| TEXAS INSTRUMENTS INCORPORATED
| Standard Linear and Logic Group
| IBIS Model of SN74LVC823A
| 9-Bit Bus-Interface Flip-Flop with 3-State Outputs
| This file contains package information for the following:
|  TSSOP 24-pin (PW) package as [Component] LVC823A_PW
|  SSOP 24-pin (DB) package as [Component] LVC823A_DB
|  TVSOP 24-pin (DGV) package as [Component] LVC823A_DGV
|  SOIC 24-pin (DW) package as [Component] LVC823A_DW
|  SOP 24-pin (NS) package as [Component] LVC823A_NS
| This device can be powered at the following Vccs:
|  1.8 volt Vcc
|  2.5 volt Vcc
|  3.3 volt Vcc
| This file provides unique models under the [Model Selector] for each Vcc.
| For operation at a specific Vcc, select the appropriate model after each
| [Model Selector] keyword.
[IBIS Ver]   3.2
[Comment char]  |_char
[File Name]   sn74lvc823a.ibs
[File Rev]   1.1 | a
[Date]   May 6, 2005
[Source]   Data created from TI-SPICE simulations at TI-SLL.
[Notes]   The following is an IBIS list for the LVC823A.
   Please contact sllibis@ti.com with questions and
   comments concerning SLL IBIS models.
   This IBIS model is created from a BA (back annotated netlist)
   - FILE REV HISTORY
   - 1.1 Release IBIS file on 05/06/05
   - Power-clamp data has been deleted since there is no
   power-clamp diode in the device.
   - Due to the fact that the device is 5-V input/output
   tolerant, the pullup data has some non-monotonic warnings.
   - End point warning due to AC and DC mismatch.
[Disclaimer] Property of Texas Instruments Incorporated.  Unauthorized
   reproduction and/or distribution is strictly prohibited.
   This product is protected under copyright law.
   Created  2005, (C) Copyright  2005, Texas Instruments
   Incorporated, All Rights Reserved
   UNLESS THERE IS A SIGNED, WRITTEN AGREEMENT TO THE
   CONTRARY, TEXAS INSTRUMENTS (TI) IS PROVIDING THE IBIS
   MODELS  AND WITHOUT ANY WARRANTY, EXPRESSED OR
   IMPLIED.  TI assumes no liability for:
   1) the accuracy of the IBIS models provided to your
   company;
   2) the proper functioning of these IBIS Models in your
   design or for any resulting applications; or
   3) infringement of patents, copyrights or intellectual
   property rights resulting from your use of these IBIS
   models.
   TI provides IBIS Models as a service to our customers.
   You and your company shall not distribute, sell or give
   these models to anyone else without prior written
   permission from TI.
   TI reserves the right to make changes to our products or
   to discontinue any semiconductor product or service
   without notice, and advises our customers to obtain the
   latest version of relevant information to verify, before
   placing orders, that the information being relied on is
   current.
   Please be aware that your receipt and use of the IBIS
   information provided shall serve as acceptance of these
   terms and conditions.  If you do not accept these terms,
   you should return or destroy the IBIS models and any
   other accompanying information immediately.
| Component LVC823A_PW 24-pin TSSOP
[Component]   LVC823A_PW
[Manufacturer]   Texas Instruments, Inc.
[Package]
|   typ   min   max
R_pkg   3.900e-02   3.000e-02   4.600e-02
L_pkg   2.685e-09   2.367e-09   3.177e-09
C_pkg   3.200e-13   2.520e-13   4.340e-13
[Pin]   signal_name   model_name   R_pin   L_pin   C_pin
1   NOE   LVC823A_NOE   3.700e-02   3.153e-09   4.340e-13
2   1D   LVC823A_IN   3.400e-02   2.629e-09   3.410e-13
3   2D   LVC823A_IN   3.200e-02   2.860e-09   3.470e-13
4   3D   LVC823A_IN   4.200e-02   2.741e-09   2.900e-13
5   4D   LVC823A_IN   4.600e-02   2.600e-09   2.620e-13
6   5D   LVC823A_IN   4.300e-02   2.414e-09   2.660e-13
7   6D   LVC823A_IN   4.200e-02   2.367e-09   2.620e-13
8   7D   LVC823A_IN   4.400e-02   2.461e-09   2.520e-13
9   8D   LVC823A_IN   4.200e-02   2.543e-09   2.740e-13
10   9D   LVC823A_IN   3.000e-02   2.616e-09   3.320e-13
11   NCLR   LVC823A_NCLR   3.700e-02   2.670e-09   3.460e-13
12   GND   GND   3.900e-02   3.177e-09   4.330e-13
13   CLK   LVC823A_CLK   3.700e-02   3.111e-09   4.310e-13
14   NCLKEN   LVC823A_NCLKEN   3.700e-02   2.656e-09   3.450e-13
15   9Q   LVC823A_OUT   3.100e-02   2.739e-09   3.400e-13
16   8Q   LVC823A_OUT   4.200e-02   2.649e-09   2.820e-13
17   7Q   LVC823A_OUT   4.600e-02   2.532e-09   2.570e-13
18   6Q   LVC823A_OUT   4.400e-02   2.425e-09   2.660e-13
19   5Q   LVC823A_OUT   4.400e-02   2.425e-09   2.660e-13
20   4Q   LVC823A_OUT   4.600e-02   2.532e-09   2.570e-13
21   3Q   LVC823A_OUT   4.200e-02   2.648e-09   2.820e-13
22   2Q   LVC823A_OUT   3.100e-02   2.738e-09   3.390e-13
23   1Q   LVC823A_OUT   3.600e-02   2.653e-09   3.440e-13
24   VCC   POWER   3.700e-02   3.110e-09   4.310e-13
| Component LVC823A_DB 24-pin SSOP
[Component]   LVC823A_DB
[Manufacturer]   Texas Instruments, Inc.
[Package]
|   typ   min   max
R_pkg   4.500e-02   4.000e-02   4.900e-02
L_pkg   3.668e-09   3.226e-09   4.415e-09
C_pkg   4.160e-13   3.490e-13   5.070e-13
[Pin]   signal_name   model_name   R_pin   L_pin   C_pin
1   NOE   LVC823A_NOE   4.200e-02   4.299e-09   5.030e-13
2   1D   LVC823A_IN   4.000e-02   3.960e-09   4.990e-13
3   2D   LVC823A_IN   4.200e-02   3.775e-09   4.170e-13
4   3D   LVC823A_IN   4.700e-02   3.487e-09   3.690e-13
5   4D   LVC823A_IN   4.600e-02   3.347e-09   3.520e-13
6   5D   LVC823A_IN   4.900e-02   3.352e-09   3.710e-13
7   6D   LVC823A_IN   4.600e-02   3.226e-09   3.630e-13
8   7D   LVC823A_IN   4.700e-02   3.289e-09   3.490e-13
9   8D   LVC823A_IN   4.700e-02   3.347e-09   3.610e-13
10   9D   LVC823A_IN   4.100e-02   3.576e-09   4.090e-13
11   NCLR   LVC823A_NCLR   4.100e-02   3.995e-09   5.030e-13
12   GND   GND   4.500e-02   4.415e-09   5.070e-13
13   CLK   LVC823A_CLK   4.300e-02   4.337e-09   5.060e-13
14   NCLKEN   LVC823A_NCLKEN   4.200e-02   4.003e-09   5.040e-13
15   9Q   LVC823A_OUT   4.100e-02   3.686e-09   4.100e-13
16   8Q   LVC823A_OUT   4.800e-02   3.355e-09   3.490e-13
17   7Q   LVC823A_OUT   4.700e-02   3.301e-09   3.530e-13
18   6Q   LVC823A_OUT   4.800e-02   3.268e-09   3.660e-13
19   5Q   LVC823A_OUT   4.800e-02   3.269e-09   3.660e-13
20   4Q   LVC823A_OUT   4.700e-02   3.314e-09   3.490e-13
21   3Q   LVC823A_OUT   4.800e-02   3.399e-09   3.550e-13
22   2Q   LVC823A_OUT   4.100e-02   3.688e-09   4.120e-13
23   1Q   LVC823A_OUT   4.200e-02   4.003e-09   5.040e-13
24   VCC   POWER   4.300e-02   4.347e-09   5.050e-13
| Component LVC823A_DGV 24-pin TVSOP
[Component]   LVC823A_DGV
[Manufacturer]   Texas Instruments, Inc.
[Package]
|   typ   min   max
R_pkg   4.300e-02   3.900e-02   4.700e-02
L_pkg   2.601e-09   2.312e-09   3.626e-09
C_pkg   3.580e-13   2.770e-13   5.950e-13
[Pin]   signal_name   model_name   R_pin   L_pin   C_pin
1   NOE   LVC823A_NOE   4.300e-02   3.625e-09   5.950e-13
2   1D   LVC823A_IN   4.000e-02   2.656e-09   4.020e-13
3   2D   LVC823A_IN   3.900e-02   2.338e-09   3.080e-13
4   3D   LVC823A_IN   4.600e-02   2.354e-09   2.770e-13
5   4D   LVC823A_IN   4.500e-02   2.312e-09   2.850e-13
6   5D   LVC823A_IN   4.700e-02   2.318e-09   2.820e-13
7   6D   LVC823A_IN   4.700e-02   2.318e-09   2.820e-13
8   7D   LVC823A_IN   4.500e-02   2.312e-09   2.850e-13
9   8D   LVC823A_IN   4.600e-02   2.353e-09   2.780e-13
10   9D   LVC823A_IN   3.900e-02   2.338e-09   3.080e-13
11   NCLR   LVC823A_NCLR   4.100e-02   2.660e-09   4.020e-13
12   GND   GND   4.300e-02   3.625e-09   5.950e-13
13   CLK   LVC823A_CLK   4.400e-02   3.626e-09   5.940e-13
14   NCLKEN   LVC823A_NCLKEN   4.000e-02   2.658e-09   4.020e-13
15   9Q   LVC823A_OUT   3.900e-02   2.343e-09   3.110e-13
16   8Q   LVC823A_OUT   4.600e-02   2.353e-09   2.780e-13
17   7Q   LVC823A_OUT   4.500e-02   2.312e-09   2.850e-13
18   6Q   LVC823A_OUT   4.700e-02   2.319e-09   2.820e-13
19   5Q   LVC823A_OUT   4.700e-02   2.319e-09   2.820e-13
20   4Q   LVC823A_OUT   4.500e-02   2.312e-09   2.850e-13
21   3Q   LVC823A_OUT   4.600e-02   2.353e-09   2.780e-13
22   2Q   LVC823A_OUT   3.900e-02   2.337e-09   3.080e-13
23   1Q   LVC823A_OUT   4.000e-02   2.658e-09   4.020e-13
24   VCC   POWER   4.400e-02   3.626e-09   5.950e-13
| Component LVC823A_DW 24-pin SOIC
[Component]   LVC823A_DW
[Manufacturer]   Texas Instruments, Inc.
[Package]
|   typ   min   max
R_pkg   3.700e-02   3.000e-02   4.700e-02
L_pkg   5.146e-09   3.993e-09   6.885e-09
C_pkg   7.580e-13   5.120e-13   1.067e-12
[Pin]   signal_name   model_name   R_pin   L_pin   C_pin
1   NOE   LVC823A_NOE   3.900e-02   6.885e-09   1.067e-12
2   D   LVC823A_IN   4.200e-02   5.950e-09   9.580e-13
3   1D   LVC823A_IN   4.700e-02   5.317e-09   7.910e-13
4   2D   LVC823A_IN   3.100e-02   4.651e-09   6.110e-13
5   3D   LVC823A_IN   3.000e-02   3.993e-09   5.120e-13
6   4D   LVC823A_IN   3.000e-02   4.083e-09   6.110e-13
7   5D   LVC823A_IN   3.000e-02   4.083e-09   6.110e-13
8   6D   LVC823A_IN   3.000e-02   3.993e-09   5.120e-13
9   7D   LVC823A_IN   3.100e-02   4.652e-09   6.110e-13
10   8D   LVC823A_IN   4.700e-02   5.317e-09   7.910e-13
11   9NCLR   LVC823A_NCLR   4.200e-02   5.950e-09   9.590e-13
12   GND   GND   3.900e-02   6.885e-09   1.067e-12
13   CLK   LVC823A_CLK   3.900e-02   6.885e-09   1.067e-12
14   NCLKEN   LVC823A_NCLKEN   4.200e-02   5.950e-09   9.590e-13
15   9Q   LVC823A_OUT   4.700e-02   5.317e-09   7.910e-13
16   8Q   LVC823A_OUT   3.100e-02   4.652e-09   6.110e-13
17   7Q   LVC823A_OUT   3.000e-02   3.993e-09   5.120e-13
18   6Q   LVC823A_OUT   3.000e-02   4.083e-09   6.100e-13
19   5Q   LVC823A_OUT   3.000e-02   4.083e-09   6.100e-13
20   4Q   LVC823A_OUT   3.000e-02   3.993e-09   5.120e-13
21   3Q   LVC823A_OUT   3.100e-02   4.651e-09   6.110e-13
22   2Q   LVC823A_OUT   4.700e-02   5.317e-09   7.910e-13
23   1Q   LVC823A_OUT   4.200e-02   5.950e-09   9.580e-13
24   VCC   POWER   3.900e-02   6.885e-09   1.067e-12
| Component LVC823A_NS 24-pin SOP
[Component]   LVC823A_NS
[Manufacturer]   Texas Instruments, Inc.
[Package]
|   typ   min   max
R_pkg   4.400e-02   3.800e-02   4.800e-02
L_pkg   3.840e-09   2.545e-09   5.234e-09
C_pkg   5.860e-13   2.740e-13   7.970e-13
[Pin]   signal_name   model_name   R_pin   L_pin   C_pin
1   NOE   LVC823A_NOE   4.100e-02   5.146e-09   7.650e-13
2   1D   LVC823A_IN   4.100e-02   4.357e-09   7.490e-13
3   2D   LVC823A_IN   4.000e-02   3.923e-09   6.330e-13
4   3D   LVC823A_IN   4.400e-02   3.412e-09   5.370e-13
5   4D   LVC823A_IN   4.500e-02   3.036e-09   3.970e-13
6   5D   LVC823A_IN   4.500e-02   2.845e-09   4.150e-13
7   6D   LVC823A_IN   4.400e-02   2.843e-09   4.150e-13
8   7D   LVC823A_IN   4.500e-02   3.065e-09   3.990e-13
9   8D   LVC823A_IN   4.500e-02   3.529e-09   5.440e-13
10   9D   LVC823A_IN   4.100e-02   4.013e-09   6.390e-13
11   NCLR   LVC823A_NCLR   4.100e-02   4.358e-09   7.460e-13
12   GND   GND   4.400e-02   5.234e-09   7.670e-13
13   CLK   LVC823A_CLK   3.900e-02   5.181e-09   7.650e-13
14   NCLKEN   LVC823A_NCLKEN   4.800e-02   4.582e-09   7.640e-13
15   9Q   LVC823A_OUT   4.100e-02   4.163e-09   6.550e-13
16   8Q   LVC823A_OUT   4.600e-02   3.613e-09   5.490e-13
17   7Q   LVC823A_OUT   4.700e-02   3.163e-09   4.060e-13
18   6Q   LVC823A_OUT   4.700e-02   2.963e-09   4.220e-13
19   5Q   LVC823A_OUT   4.700e-02   2.919e-09   4.190e-13
20   4Q   LVC823A_OUT   4.800e-02   3.087e-09   4.870e-13
21   3Q   LVC823A_OUT   4.600e-02   4.513e-09   7.600e-13
22   2Q   LVC823A_OUT   4.200e-02   4.505e-09   7.670e-13
23   1Q   LVC823A_OUT   4.200e-02   5.163e-09   7.970e-13
24   VCC   POWER   3.800e-02   2.545e-09   2.740e-13
| Model LVC823A_NOE
[Model Selector]   LVC823A_NOE
LVC823A_NOE_18   1.8 volt Vcc
LVC823A_NOE_25   2.5 volt Vcc
LVC823A_NOE_33   3.3 volt Vcc
| Model LVC823A_NCLR
[Model Selector]   LVC823A_NCLR
LVC823A_NCLR_18   1.8 volt Vcc
LVC823A_NCLR_25   2.5 volt Vcc
LVC823A_NCLR_33   3.3 volt Vcc
| Model LVC823A_NCLKEN
[Model Selector]   LVC823A_NCLKEN
LVC823A_NCLKEN_18   1.8 volt Vcc
LVC823A_NCLKEN_25   2.5 volt Vcc
LVC823A_NCLKEN_33   3.3 volt Vcc
| Model LVC823A_CLK
[Model Selector]   LVC823A_CLK
LVC823A_CLK_18   1.8 volt Vcc
LVC823A_CLK_25   2.5 volt Vcc
LVC823A_CLK_33   3.3 volt Vcc
| Model LVC823A_IN
[Model Selector]   LVC823A_IN
LVC823A_IN_18   1.8 volt Vcc
LVC823A_IN_25   2.5 volt Vcc
LVC823A_IN_33   3.3 volt Vcc
| Model LVC823A_OUT
[Model Selector]   LVC823A_OUT
LVC823A_OUT_18   1.8 volt Vcc
LVC823A_OUT_25   2.5 volt Vcc
LVC823A_OUT_33   3.3 volt Vcc
| Models and submodels in the file (18): LVC823A_NOE_18 (Input), LVC823A_NOE_25 (Input), LVC823A_NOE_33 (Input), LVC823A_NCLR_18 (Input), LVC823A_NCLR_25 (Input), LVC823A_NCLR_33 (Input), LVC823A_NCLKEN_18 (Input), LVC823A_NCLKEN_25 (Input), LVC823A_NCLKEN_33 (Input), LVC823A_CLK_18 (Input), LVC823A_CLK_25 (Input), LVC823A_CLK_33 (Input), LVC823A_IN_18 (Input), LVC823A_IN_25 (Input), LVC823A_IN_33 (Input), LVC823A_OUT_18 (3-state), LVC823A_OUT_25 (3-state), LVC823A_OUT_33 (3-state)
